(* Logix 5000 Routine export FMSExample; software revision 24.00 *)

TYPE FFLinkFMSResponse :
STRUCT
   Status : INT;   // 0=Success, 1=Timeout, 2=DLSeqMismatch, 3=InvokeIDMismatch, 4=FMSError
   DataLength : INT;
   CallBackID : DINT;
   Data : SINT[32];
END_STRUCT
END_TYPE

TYPE FFLinkFMSRequest :
STRUCT
   StationAddress : SINT;
   VFDSelector : SINT;   // 0=System, 1=AP
   Command : SINT;   // 0=Reserved, 1=Read, 2=Write
   CallBackID : DINT;
   TimeOut : INT;   // Timeout in milliseconds
   Index : INT;
   SubIndex : INT;
   DataLength : INT;
   Data : SINT[32];
END_STRUCT
END_TYPE

TYPE FFLinkFMSService :
STRUCT
   Request : FFLinkFMSRequest;
   Response : FFLinkFMSResponse;
END_STRUCT
END_TYPE

ADD_ON_INSTRUCTION FFLinkFMSGeneralRW   (* revision 1.0, vendor Aparian *)
VAR_INPUT
   StationAddress : INT; {required}
   Command : INT; {required}
   BlockIndex : INT; {required}
   Index : INT; {required}
   SubIndex : INT; {required}
   TimeOut : INT; {required}
   RequestDataLength : INT; {required}
   ResponseDataLength : INT; {required}
END_VAR
VAR_IN_OUT
   FMS : FFLinkFMSService; {required}
   Msg : MESSAGE; {required}
END_VAR
VAR_OUTPUT
   Busy : BOOL; {access Read Only, required}
   Success : BOOL; {access Read Only, required}
   Fail : BOOL; {access Read Only, required}
   MsgError : BOOL; {access Read Only, required}
   TimeOutErr : BOOL; {access Read Only, required}
   DataLinkErr : BOOL; {access Read Only, required}
   FMSError : BOOL; {access Read Only, required}
   Status : INT; {access Read Only, required}
   FMSErrorCode : DINT; {access Read Only, required}
   StatusOk : BOOL; {access Read Only, visible}
   ProcessData : BOOL; {visible}
END_VAR

ROUTINE Logic   (* ladder *)
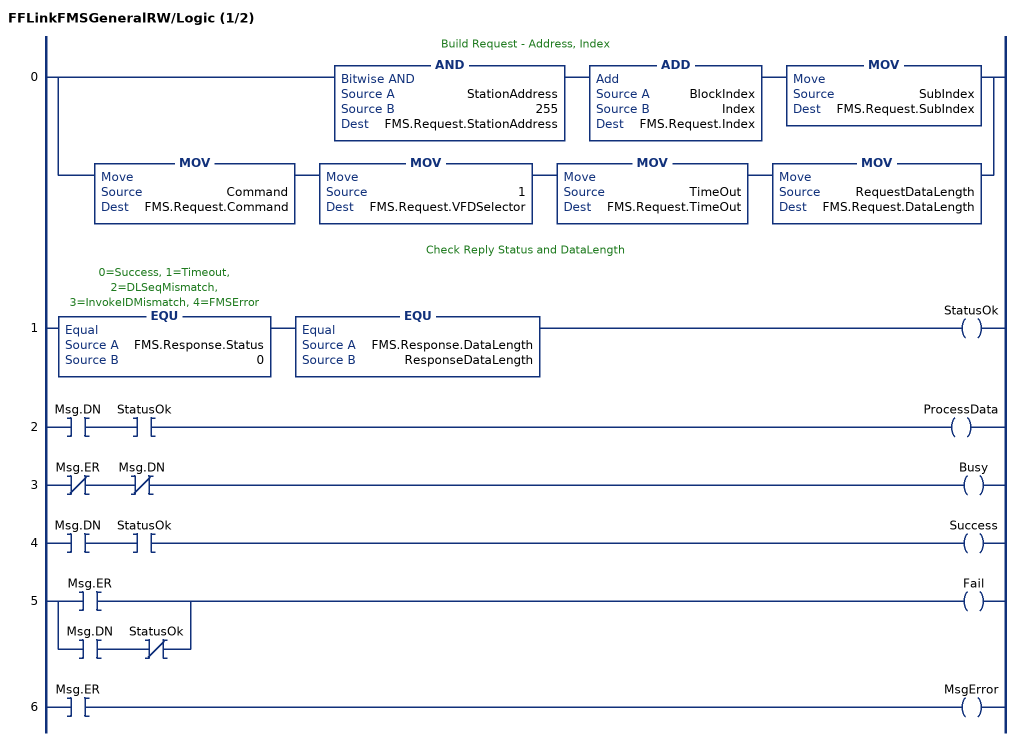
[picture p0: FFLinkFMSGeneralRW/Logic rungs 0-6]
   // Build Request - Address, Index
   0: [AND(StationAddress,255,FMS.Request.StationAddress) ADD(BlockIndex,Index,FMS.Request.Index) MOV(SubIndex,FMS.Request.SubIndex) ,MOV(Command,FMS.Request.Command) MOV(1,FMS.Request.VFDSelector) MOV(TimeOut,FMS.Request.TimeOut) MOV(RequestDataLength,FMS.Request.DataLength) ];
   // Check Reply Status and DataLength
   1: EQU(FMS.Response.Status,0)EQU(FMS.Response.DataLength,ResponseDataLength)OTE(StatusOk);
   2: XIC(Msg.DN)XIC(StatusOk)OTE(ProcessData);
   3: XIO(Msg.ER)XIO(Msg.DN)OTE(Busy);
   4: XIC(Msg.DN)XIC(StatusOk)OTE(Success);
   5: [XIC(Msg.ER) ,XIC(Msg.DN) XIO(StatusOk) ]OTE(Fail);
   6: XIC(Msg.ER)OTE(MsgError);
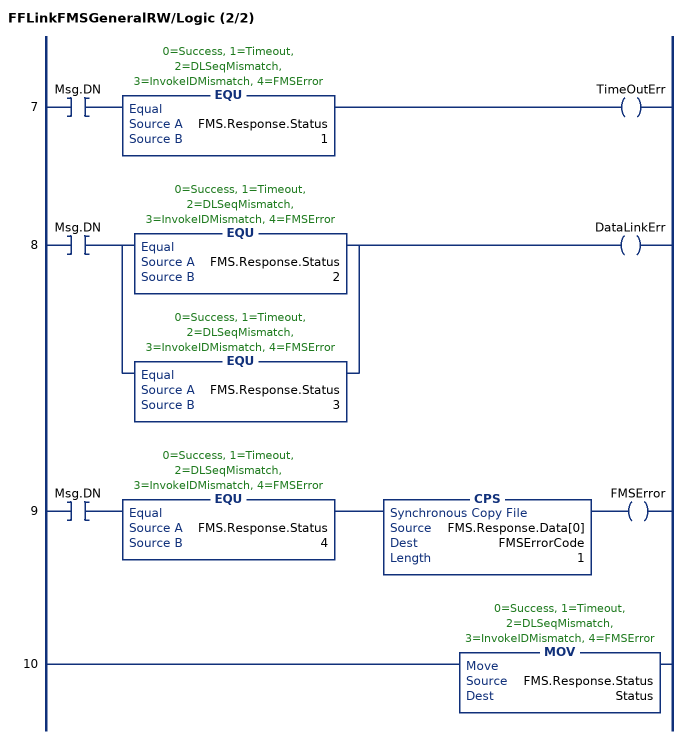
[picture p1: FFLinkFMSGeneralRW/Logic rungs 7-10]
   7: XIC(Msg.DN)EQU(FMS.Response.Status,1)OTE(TimeOutErr);
   8: XIC(Msg.DN)[EQU(FMS.Response.Status,2) ,EQU(FMS.Response.Status,3) ]OTE(DataLinkErr);
   9: XIC(Msg.DN)EQU(FMS.Response.Status,4)CPS(FMS.Response.Data[0],FMSErrorCode,1)OTE(FMSError);
   10: MOV(FMS.Response.Status,Status);
END_ROUTINE
END_ADD_ON_INSTRUCTION

ADD_ON_INSTRUCTION FFLinkFMSReadDINT   (* revision 1.0, vendor Aparian *)
VAR_INPUT
   StationAddress : INT; {required}
   BlockIndex : INT; {required}
   Index : INT; {required}
   SubIndex : INT; {required}
   TimeOut : INT; {required}
END_VAR
VAR_OUTPUT
   ReadValue : DINT; {access Read Only, required}
END_VAR
VAR_IN_OUT
   FMS : FFLinkFMSService; {required}
   Msg : MESSAGE; {required}
END_VAR
VAR_OUTPUT
   Busy : BOOL; {access Read Only, visible}
   Success : BOOL; {access Read Only, visible}
   Fail : BOOL; {access Read Only, visible}
   MsgError : BOOL; {access Read Only, visible}
   TimeOutErr : BOOL; {access Read Only, visible}
   DataLinkErr : BOOL; {access Read Only, visible}
   FMSError : BOOL; {access Read Only, visible}
   Status : INT; {access Read Only}
   FMSErrorCode : DINT; {access Read Only}
END_VAR
VAR
   tempDINT : DINT; {access None}
   GeneralRW : FFLinkFMSGeneralRW; {access None}
END_VAR

ROUTINE Logic   (* ladder *)
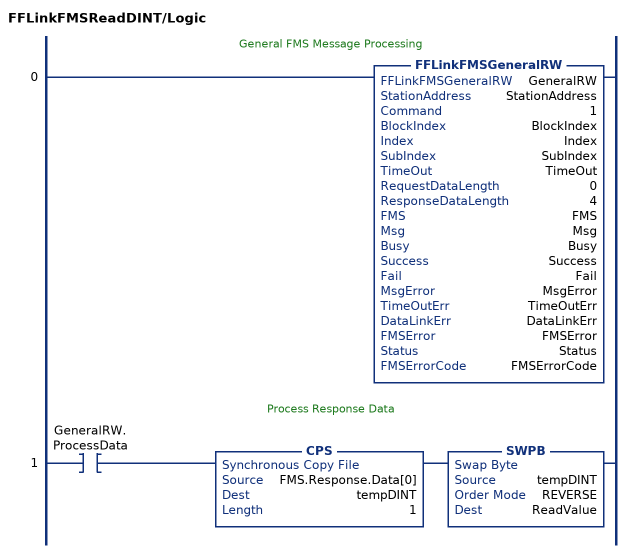
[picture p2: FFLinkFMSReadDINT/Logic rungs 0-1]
   // General FMS Message Processing
   0: FFLinkFMSGeneralRW(GeneralRW,StationAddress,1,BlockIndex,Index,SubIndex,TimeOut,0,4,FMS,Msg,Busy,Success,Fail,MsgError,TimeOutErr,DataLinkErr,FMSError,Status,FMSErrorCode);
   // Process Response Data
   1: XIC(GeneralRW.ProcessData)CPS(FMS.Response.Data[0],tempDINT,1)SWPB(tempDINT,REVERSE,ReadValue);
END_ROUTINE
END_ADD_ON_INSTRUCTION

ADD_ON_INSTRUCTION FFLinkFMSReadINT   (* revision 1.0, vendor Aparian *)
VAR_INPUT
   StationAddress : INT; {required}
   BlockIndex : INT; {required}
   Index : INT; {required}
   SubIndex : INT; {required}
   TimeOut : INT; {required}
END_VAR
VAR_OUTPUT
   ReadValue : INT; {access Read Only, required}
END_VAR
VAR_IN_OUT
   FMS : FFLinkFMSService; {required}
   Msg : MESSAGE; {required}
END_VAR
VAR_OUTPUT
   Busy : BOOL; {access Read Only, visible}
   Success : BOOL; {access Read Only, visible}
   Fail : BOOL; {access Read Only, visible}
   MsgError : BOOL; {access Read Only, visible}
   TimeOutErr : BOOL; {access Read Only, visible}
   DataLinkErr : BOOL; {access Read Only, visible}
   FMSError : BOOL; {access Read Only, visible}
   Status : INT; {access Read Only}
   FMSErrorCode : DINT; {access Read Only}
END_VAR
VAR
   tempINT : INT; {access None}
   GeneralRW : FFLinkFMSGeneralRW; {access None}
END_VAR

ROUTINE Logic   (* ladder *)
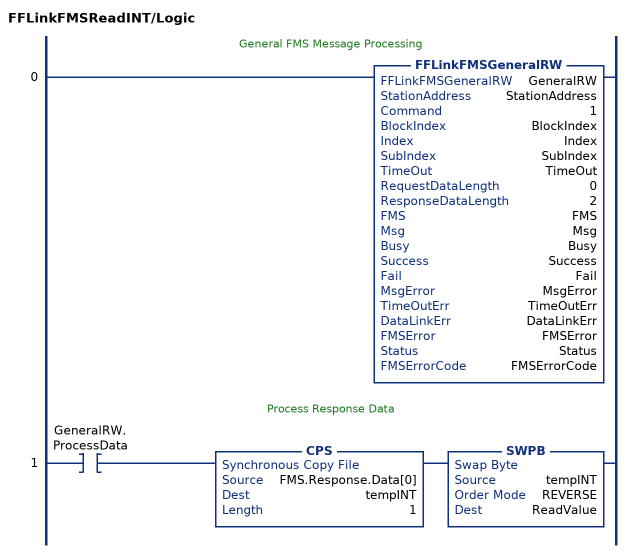
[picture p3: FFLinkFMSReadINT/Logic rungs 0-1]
   // General FMS Message Processing
   0: FFLinkFMSGeneralRW(GeneralRW,StationAddress,1,BlockIndex,Index,SubIndex,TimeOut,0,2,FMS,Msg,Busy,Success,Fail,MsgError,TimeOutErr,DataLinkErr,FMSError,Status,FMSErrorCode);
   // Process Response Data
   1: XIC(GeneralRW.ProcessData)CPS(FMS.Response.Data[0],tempINT,1)SWPB(tempINT,REVERSE,ReadValue);
END_ROUTINE
END_ADD_ON_INSTRUCTION

ADD_ON_INSTRUCTION FFLinkFMSReadREAL   (* revision 1.0, vendor Aparian *)
VAR_INPUT
   StationAddress : INT; {required}
   BlockIndex : INT; {required}
   Index : INT; {required}
   SubIndex : INT; {required}
   TimeOut : INT; {required}
END_VAR
VAR_OUTPUT
   ReadValue : REAL; {access Read Only, required}
END_VAR
VAR_IN_OUT
   FMS : FFLinkFMSService; {required}
   Msg : MESSAGE; {required}
END_VAR
VAR_OUTPUT
   Busy : BOOL; {access Read Only, visible}
   Success : BOOL; {access Read Only, visible}
   Fail : BOOL; {access Read Only, visible}
   MsgError : BOOL; {access Read Only, visible}
   TimeOutErr : BOOL; {access Read Only, visible}
   DataLinkErr : BOOL; {access Read Only, visible}
   FMSError : BOOL; {access Read Only, visible}
   Status : INT; {access Read Only}
   FMSErrorCode : DINT; {access Read Only}
END_VAR
VAR
   tempREAL : REAL; {access None}
   GeneralRW : FFLinkFMSGeneralRW; {access None}
   tempDINT : DINT; {access None}
   tempDINT2 : DINT; {access None}
END_VAR

ROUTINE Logic   (* ladder *)
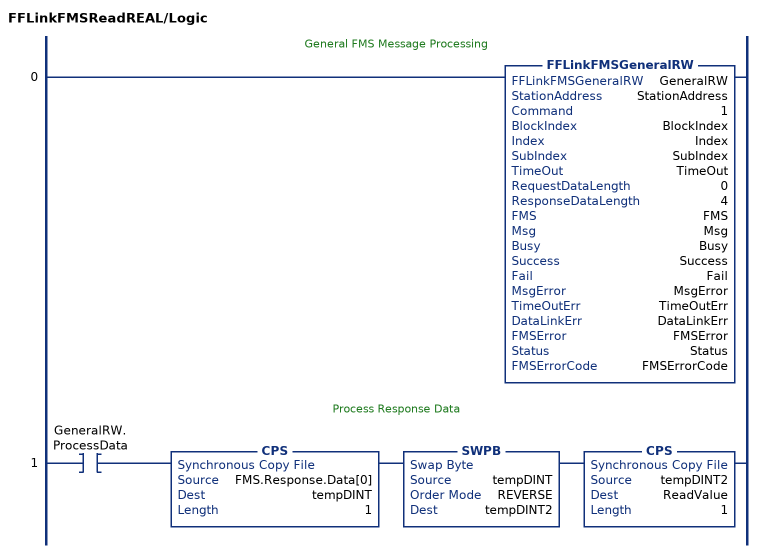
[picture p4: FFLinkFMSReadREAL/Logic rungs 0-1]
   // General FMS Message Processing
   0: FFLinkFMSGeneralRW(GeneralRW,StationAddress,1,BlockIndex,Index,SubIndex,TimeOut,0,4,FMS,Msg,Busy,Success,Fail,MsgError,TimeOutErr,DataLinkErr,FMSError,Status,FMSErrorCode);
   // Process Response Data
   1: XIC(GeneralRW.ProcessData)CPS(FMS.Response.Data[0],tempDINT,1)SWPB(tempDINT,REVERSE,tempDINT2)CPS(tempDINT2,ReadValue,1);
END_ROUTINE
END_ADD_ON_INSTRUCTION

ADD_ON_INSTRUCTION FFLinkFMSReadSINT   (* revision 1.0, vendor Aparian *)
VAR_INPUT
   StationAddress : INT; {required}
   BlockIndex : INT; {required}
   Index : INT; {required}
   SubIndex : INT; {required}
   TimeOut : INT; {required}
END_VAR
VAR_OUTPUT
   ReadValue : SINT; {access Read Only, required}
END_VAR
VAR_IN_OUT
   FMS : FFLinkFMSService; {required}
   Msg : MESSAGE; {required}
END_VAR
VAR_OUTPUT
   Busy : BOOL; {access Read Only, visible}
   Success : BOOL; {access Read Only, visible}
   Fail : BOOL; {access Read Only, visible}
   MsgError : BOOL; {access Read Only, visible}
   TimeOutErr : BOOL; {access Read Only, visible}
   DataLinkErr : BOOL; {access Read Only, visible}
   FMSError : BOOL; {access Read Only, visible}
   Status : INT; {access Read Only}
   FMSErrorCode : DINT; {access Read Only}
END_VAR
VAR
   GeneralRW : FFLinkFMSGeneralRW; {access None}
END_VAR

ROUTINE Logic   (* ladder *)
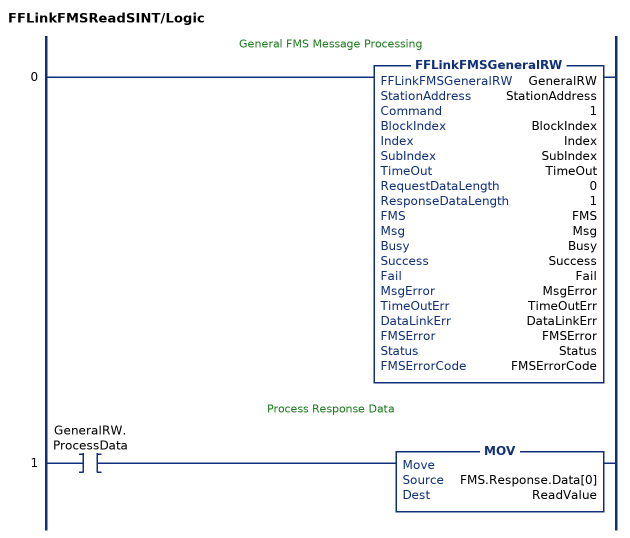
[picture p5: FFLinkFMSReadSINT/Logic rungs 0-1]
   // General FMS Message Processing
   0: FFLinkFMSGeneralRW(GeneralRW,StationAddress,1,BlockIndex,Index,SubIndex,TimeOut,0,1,FMS,Msg,Busy,Success,Fail,MsgError,TimeOutErr,DataLinkErr,FMSError,Status,FMSErrorCode);
   // Process Response Data
   1: XIC(GeneralRW.ProcessData)MOV(FMS.Response.Data[0],ReadValue);
END_ROUTINE
END_ADD_ON_INSTRUCTION

ADD_ON_INSTRUCTION FFLinkFMSWriteDINT   (* revision 1.0, vendor Aparian *)
VAR_INPUT
   StationAddress : INT; {required}
   BlockIndex : INT; {required}
   Index : INT; {required}
   SubIndex : INT; {required}
   TimeOut : INT; {required}
   WriteValue : DINT; {required}
END_VAR
VAR_IN_OUT
   FMS : FFLinkFMSService; {required}
   Msg : MESSAGE; {required}
END_VAR
VAR_OUTPUT
   Busy : BOOL; {access Read Only, visible}
   Success : BOOL; {access Read Only, visible}
   Fail : BOOL; {access Read Only, visible}
   MsgError : BOOL; {access Read Only, visible}
   TimeOutErr : BOOL; {access Read Only, visible}
   DataLinkErr : BOOL; {access Read Only, visible}
   FMSError : BOOL; {access Read Only, visible}
   Status : INT; {access Read Only}
   FMSErrorCode : DINT; {access Read Only}
END_VAR
VAR
   tempDINT : DINT; {access None}
   GeneralRW : FFLinkFMSGeneralRW; {access None}
END_VAR

ROUTINE Logic   (* ladder *)
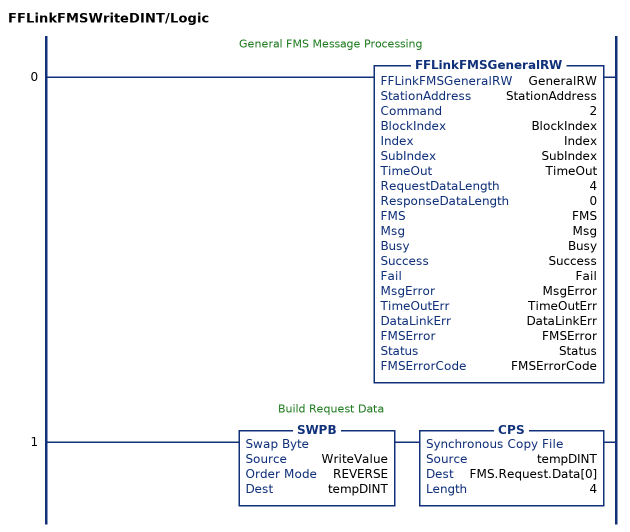
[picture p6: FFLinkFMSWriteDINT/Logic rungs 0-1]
   // General FMS Message Processing
   0: FFLinkFMSGeneralRW(GeneralRW,StationAddress,2,BlockIndex,Index,SubIndex,TimeOut,4,0,FMS,Msg,Busy,Success,Fail,MsgError,TimeOutErr,DataLinkErr,FMSError,Status,FMSErrorCode);
   // Build Request Data
   1: SWPB(WriteValue,REVERSE,tempDINT)CPS(tempDINT,FMS.Request.Data[0],4);
END_ROUTINE
END_ADD_ON_INSTRUCTION

ADD_ON_INSTRUCTION FFLinkFMSWriteINT   (* revision 1.0, vendor Aparian *)
VAR_INPUT
   StationAddress : INT; {required}
   BlockIndex : INT; {required}
   Index : INT; {required}
   SubIndex : INT; {required}
   TimeOut : INT; {required}
   WriteValue : INT; {required}
END_VAR
VAR_IN_OUT
   FMS : FFLinkFMSService; {required}
   Msg : MESSAGE; {required}
END_VAR
VAR_OUTPUT
   Busy : BOOL; {access Read Only, visible}
   Success : BOOL; {access Read Only, visible}
   Fail : BOOL; {access Read Only, visible}
   MsgError : BOOL; {access Read Only, visible}
   TimeOutErr : BOOL; {access Read Only, visible}
   DataLinkErr : BOOL; {access Read Only, visible}
   FMSError : BOOL; {access Read Only, visible}
   Status : INT; {access Read Only}
   FMSErrorCode : DINT; {access Read Only}
END_VAR
VAR
   tempINT : INT; {access None}
   GeneralRW : FFLinkFMSGeneralRW; {access None}
END_VAR

ROUTINE Logic   (* ladder *)
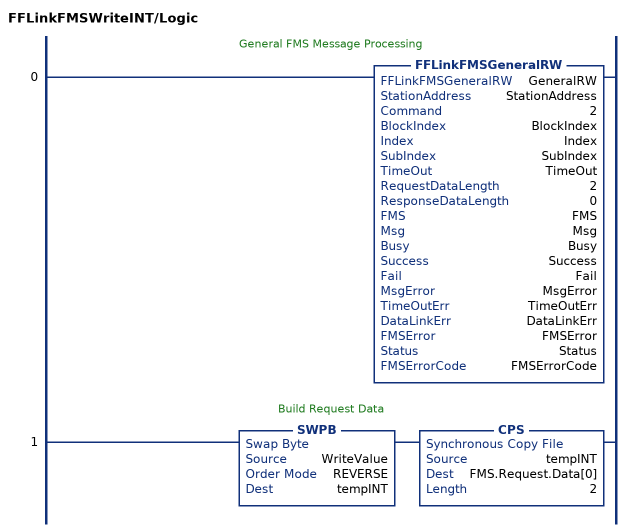
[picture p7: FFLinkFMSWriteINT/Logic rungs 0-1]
   // General FMS Message Processing
   0: FFLinkFMSGeneralRW(GeneralRW,StationAddress,2,BlockIndex,Index,SubIndex,TimeOut,2,0,FMS,Msg,Busy,Success,Fail,MsgError,TimeOutErr,DataLinkErr,FMSError,Status,FMSErrorCode);
   // Build Request Data
   1: SWPB(WriteValue,REVERSE,tempINT)CPS(tempINT,FMS.Request.Data[0],2);
END_ROUTINE
END_ADD_ON_INSTRUCTION

ADD_ON_INSTRUCTION FFLinkFMSWriteREAL   (* revision 1.0, vendor Aparian *)
VAR_INPUT
   StationAddress : INT; {required}
   BlockIndex : INT; {required}
   Index : INT; {required}
   SubIndex : INT; {required}
   TimeOut : INT; {required}
   WriteValue : REAL; {required}
END_VAR
VAR_IN_OUT
   FMS : FFLinkFMSService; {required}
   Msg : MESSAGE; {required}
END_VAR
VAR_OUTPUT
   Busy : BOOL; {access Read Only, visible}
   Success : BOOL; {access Read Only, visible}
   Fail : BOOL; {access Read Only, visible}
   MsgError : BOOL; {access Read Only, visible}
   TimeOutErr : BOOL; {access Read Only, visible}
   DataLinkErr : BOOL; {access Read Only, visible}
   FMSError : BOOL; {access Read Only, visible}
   Status : INT; {access Read Only}
   FMSErrorCode : DINT; {access Read Only}
END_VAR
VAR
   tempREAL : REAL; {access None}
   GeneralRW : FFLinkFMSGeneralRW; {access None}
   tempDINT : DINT; {access None}
   tempDINT2 : DINT; {access None}
END_VAR

ROUTINE Logic   (* ladder *)
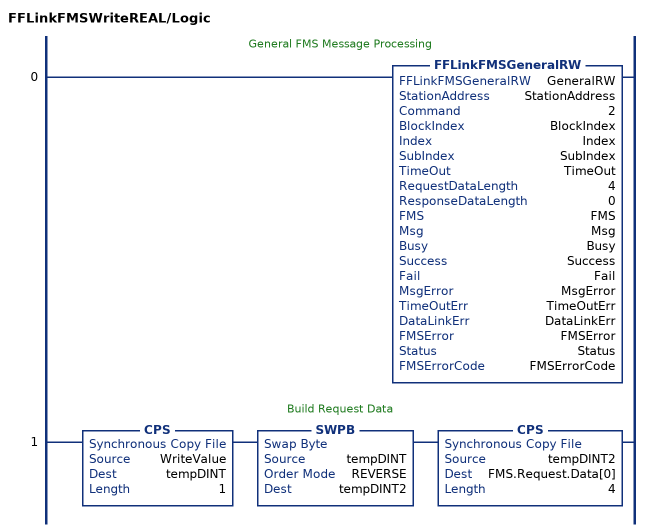
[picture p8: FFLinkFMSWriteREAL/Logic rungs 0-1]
   // General FMS Message Processing
   0: FFLinkFMSGeneralRW(GeneralRW,StationAddress,2,BlockIndex,Index,SubIndex,TimeOut,4,0,FMS,Msg,Busy,Success,Fail,MsgError,TimeOutErr,DataLinkErr,FMSError,Status,FMSErrorCode);
   // Build Request Data
   1: CPS(WriteValue,tempDINT,1)SWPB(tempDINT,REVERSE,tempDINT2)CPS(tempDINT2,FMS.Request.Data[0],4);
END_ROUTINE
END_ADD_ON_INSTRUCTION

ADD_ON_INSTRUCTION FFLinkFMSWriteSINT   (* revision 1.0, vendor Aparian *)
VAR_INPUT
   StationAddress : INT; {required}
   BlockIndex : INT; {required}
   Index : INT; {required}
   SubIndex : INT; {required}
   TimeOut : INT; {required}
   WriteValue : SINT; {required}
END_VAR
VAR_IN_OUT
   FMS : FFLinkFMSService; {required}
   Msg : MESSAGE; {required}
END_VAR
VAR_OUTPUT
   Busy : BOOL; {access Read Only, visible}
   Success : BOOL; {access Read Only, visible}
   Fail : BOOL; {access Read Only, visible}
   MsgError : BOOL; {access Read Only, visible}
   TimeOutErr : BOOL; {access Read Only, visible}
   DataLinkErr : BOOL; {access Read Only, visible}
   FMSError : BOOL; {access Read Only, visible}
   Status : INT; {access Read Only}
   FMSErrorCode : DINT; {access Read Only}
END_VAR
VAR
   tempSINT : SINT; {access None}
   GeneralRW : FFLinkFMSGeneralRW; {access None}
END_VAR

ROUTINE Logic   (* ladder *)
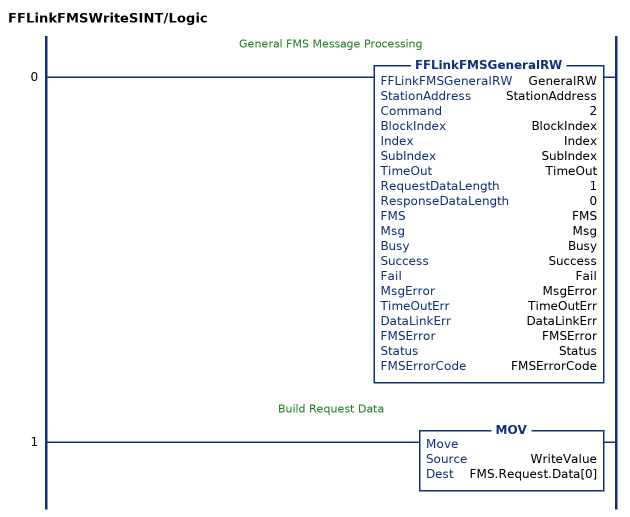
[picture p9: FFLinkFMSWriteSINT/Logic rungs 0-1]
   // General FMS Message Processing
   0: FFLinkFMSGeneralRW(GeneralRW,StationAddress,2,BlockIndex,Index,SubIndex,TimeOut,1,0,FMS,Msg,Busy,Success,Fail,MsgError,TimeOutErr,DataLinkErr,FMSError,Status,FMSErrorCode);
   // Build Request Data
   1: MOV(WriteValue,FMS.Request.Data[0]);
END_ROUTINE
END_ADD_ON_INSTRUCTION

VAR_GLOBAL   (* controller tags *)
   FMSCtrl001 : FFLinkFMSWriteREAL := (StationAddress := 55, BlockIndex := 1000, Index := 8, SubIndex := 8, TimeOut := 2000, WriteValue := 27.7, Success := 1);
   TestValue001 : REAL := 27.7;
   FMSMsg001 : MESSAGE;
        MessageParameters(MessageType := CIP Generic, RequestedLength := 32, ConnectedFlag := 2, ConnectionPath := FFL01, ServiceCode := 16#0066, ObjectType := 16#0434, TargetObject := 1, LocalElement := FMS001.Request, DestinationTag := FMS001.Response)
   FMS001 : FFLinkFMSService := (Request.StationAddress := 55, Request.VFDSelector := 1, Request.Command := 2, Request.TimeOut := 2000, Request.Index := 1008, Request.SubIndex := 8, Request.DataLength := 4, Request.Data[0] := 65, Request.Data[1] := -35, Request.Data[2] := -103, Request.Data[3] := -102, Response.Data[0] := -127, Response.Data[1] := 97, Response.Data[2] := 7);
   Test001 : BOOL := 1;
END_VAR

PROGRAM MainProgram

ROUTINE FMSExample   (* ladder *)
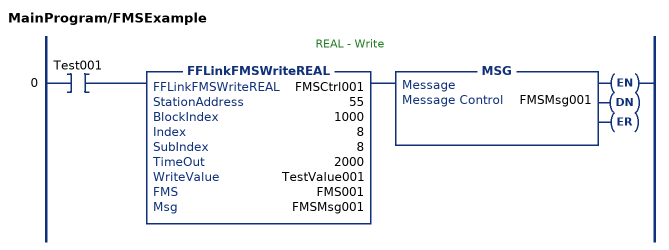
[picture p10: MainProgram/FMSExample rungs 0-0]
   // REAL - Write
   0: XIC(Test001)FFLinkFMSWriteREAL(FMSCtrl001,55,1000,8,8,2000,TestValue001,FMS001,FMSMsg001)MSG(FMSMsg001);
END_ROUTINE
END_PROGRAM
